(* Logix 5000 Rung export; software revision 33.00 *)

TYPE Banner_IOL_Device_Index_v6 :
STRUCT
   Index : Banner_IOL_Device_SubIndex_v6[41];
END_STRUCT
END_TYPE

TYPE Banner_IOL_Device_SubIndex_v6 :
STRUCT
   Sub : DINT[34];
END_STRUCT
END_TYPE

TYPE Banner_IOL_Device_v6 :
STRUCT
   Initial_Global_Read : BOOL;
   Command : SINT;
   Data : Banner_IOL_Device_Index_v6;
   Reset : BOOL;
END_STRUCT
END_TYPE

TYPE Banner_IOL_Rules_Array_v6 :
STRUCT
   Length : DINT;
   Settings : Banner_IOL_Rules_SettingsArray_v6[41];
END_STRUCT
END_TYPE

TYPE Banner_IOL_Rules_SettingsArray_v6 :
STRUCT
   Index : DINT;
   Sub_Index : DINT;
   Num_Op : INT;   // Number of Operations to read/write Index.
   Total_Bytes : INT;
   RW : SINT;   // 0 = Read Only, 1 = Write Only, 2 = Read or Write
   Rules : Banner_IOL_Rules_v6[34];   // Sub Index Position in IODD.
END_STRUCT
END_TYPE

TYPE Banner_IOL_Rules_v6 :
STRUCT
   Byte_Pos : SINT;   // Byte Position to read from or write data to.
   Multi : SINT;   // Determines if a multiple byte length index is being accessed. Use 2 for 2 bytes length, 3 for 3 byte length, etc..
   BitControl : BOOL;   // 0=Standard byte control, 1=Bitwise packaging
   BitPos : SINT;   // Bit start position for operation
   BitValue : SINT;
   Sub_Index : SINT;
   Signed : SINT;   // 0=Unsigned, 1=Signed
END_STRUCT
END_TYPE

VAR_GLOBAL   (* controller tags *)
   TL70PS_IOLM1_01 : Banner_IOL_Device_v6;
        .DATA.INDEX[2]   // Direct Parameters 1
        .DATA.INDEX[2].SUB[1]   // Reserved
        .DATA.INDEX[2].SUB[2]   // Master Cycle Time
        .DATA.INDEX[2].SUB[3]   // Min Cycle Time
        .DATA.INDEX[2].SUB[4]   // M Sequence Capability
        .DATA.INDEX[2].SUB[5]   // IO-Link Verson ID
        .DATA.INDEX[2].SUB[6]   // Process Data Input Length
        .DATA.INDEX[2].SUB[7]   // Process Data Output Length
        .DATA.INDEX[2].SUB[8]   // Vendor ID
        .DATA.INDEX[2].SUB[9]   // Device ID
        .DATA.INDEX[3]   // Standard Command (wo)
        .DATA.INDEX[3].SUB[1]   // Standard Command: 130=Restore Factory Settings
        .DATA.INDEX[4]   // Device Locks
        .DATA.INDEX[4].SUB[1]   // Parameter Access Lock: 0 to 1
        .DATA.INDEX[4].SUB[2]   // Data Storage Lock: 0 to 1
        .DATA.INDEX[4].SUB[3]   // Local Parameterization Lock: 0 to 1
        .DATA.INDEX[4].SUB[4]   // Local User Interface Lock: 0 to 1
        .DATA.INDEX[5]   // Serial Number (ro)
        .DATA.INDEX[5].SUB[1]   // SN1
        .DATA.INDEX[5].SUB[2]   // SN2
        .DATA.INDEX[5].SUB[3]   // SN3
        .DATA.INDEX[5].SUB[4]   // SN4
        .DATA.INDEX[5].SUB[5]   // SN5
        .DATA.INDEX[5].SUB[6]   // SN6
        .DATA.INDEX[5].SUB[7]   // SN7
        .DATA.INDEX[5].SUB[8]   // SN8
        .DATA.INDEX[5].SUB[9]   // SN9
        .DATA.INDEX[5].SUB[10]   // SN10
        .DATA.INDEX[5].SUB[11]   // SN11
        .DATA.INDEX[5].SUB[12]   // SN12
        .DATA.INDEX[5].SUB[13]   // SN13
        .DATA.INDEX[5].SUB[14]   // SN14
        .DATA.INDEX[5].SUB[15]   // SN15
        .DATA.INDEX[5].SUB[16]   // SN16
        .DATA.INDEX[6]   // Operating Mode Selection
        .DATA.INDEX[6].SUB[1]   // Operating Mode Selection: 0=Basic Segment Mode, 1=Run Mode, 2=Advanced Segment Mode, 3=Level Mode
        .DATA.INDEX[7]   // Segment 1 Configuration
        .DATA.INDEX[7].SUB[1]   // Animation: 0=Off, 1=Steady, 2=Flash, 3=Two Color Flash, 4=Half/Half, 5=Half/Half Rotate, 6=Chase, 7=Intensity Sweep, 8=Demo
        .DATA.INDEX[7].SUB[2]   // Color 1: 0=Green, 1=Red, 2=Orange, 3=Amber, 4=Yellow, 5=Lime Green, 6=Spring Green, 7=Cyan, 8=Sky Blue, 9=Blue, 10=Violet, 11=Magenta, 12=Rose, 13=White
        .DATA.INDEX[7].SUB[3]   // Color 2: 0=Green, 1=Red, 2=Orange, 3=Amber, 4=Yellow, 5=Lime Green, 6=Spring Green, 7=Cyan, 8=Sky Blue, 9=Blue, 10=Violet, 11=Magenta, 12=Rose, 13=White
        .DATA.INDEX[7].SUB[4]   // Color 1 Intensity: 0=High, 1=Medium, 2=Low, 3=Off, 4=Custom
        .DATA.INDEX[7].SUB[5]   // Color 2 Intensity: 0=High, 1=Medium, 2=Low, 3=Off, 4=Custom
        .DATA.INDEX[7].SUB[6]   // Speed: 0=Medium, 1=Slow, 2=Fast, 3=Custom
        .DATA.INDEX[7].SUB[7]   // Pattern: 0=Flash, 1=Strobe, 2=3 Pulse, 3=SOS, 4=Random
        .DATA.INDEX[8]   // Segment 2 Configuration
        .DATA.INDEX[8].SUB[1]   // Animation: 0=Off, 1=Steady, 2=Flash, 3=Two Color Flash, 4=Half/Half, 5=Half/Half Rotate, 6=Chase, 7=Intensity Sweep, 8=Demo
        .DATA.INDEX[8].SUB[2]   // Color 1: 0=Green, 1=Red, 2=Orange, 3=Amber, 4=Yellow, 5=Lime Green, 6=Spring Green, 7=Cyan, 8=Sky Blue, 9=Blue, 10=Violet, 11=Magenta, 12=Rose, 13=White
        .DATA.INDEX[8].SUB[3]   // Color 2: 0=Green, 1=Red, 2=Orange, 3=Amber, 4=Yellow, 5=Lime Green, 6=Spring Green, 7=Cyan, 8=Sky Blue, 9=Blue, 10=Violet, 11=Magenta, 12=Rose, 13=White
        .DATA.INDEX[8].SUB[4]   // Color 1 Intensity: 0=High, 1=Medium, 2=Low, 3=Off, 4=Custom
        .DATA.INDEX[8].SUB[5]   // Color 2 Intensity: 0=High, 1=Medium, 2=Low, 3=Off, 4=Custom
        .DATA.INDEX[8].SUB[6]   // Speed: 0=Medium, 1=Slow, 2=Fast, 3=Custom
        .DATA.INDEX[8].SUB[7]   // Pattern: 0=Flash, 1=Strobe, 2=3 Pulse, 3=SOS, 4=Random
        .DATA.INDEX[9]   // Segment 3 Configuration
        .DATA.INDEX[9].SUB[1]   // Animation: 0=Off, 1=Steady, 2=Flash, 3=Two Color Flash, 4=Half/Half, 5=Half/Half Rotate, 6=Chase, 7=Intensity Sweep, 8=Demo
        .DATA.INDEX[9].SUB[2]   // Color 1: 0=Green, 1=Red, 2=Orange, 3=Amber, 4=Yellow, 5=Lime Green, 6=Spring Green, 7=Cyan, 8=Sky Blue, 9=Blue, 10=Violet, 11=Magenta, 12=Rose, 13=White
        .DATA.INDEX[9].SUB[3]   // Color 2: 0=Green, 1=Red, 2=Orange, 3=Amber, 4=Yellow, 5=Lime Green, 6=Spring Green, 7=Cyan, 8=Sky Blue, 9=Blue, 10=Violet, 11=Magenta, 12=Rose, 13=White
        .DATA.INDEX[9].SUB[4]   // Color 1 Intensity: 0=High, 1=Medium, 2=Low, 3=Off, 4=Custom
        .DATA.INDEX[9].SUB[5]   // Color 2 Intensity: 0=High, 1=Medium, 2=Low, 3=Off, 4=Custom
        .DATA.INDEX[9].SUB[6]   // Speed: 0=Medium, 1=Slow, 2=Fast, 3=Custom
        .DATA.INDEX[9].SUB[7]   // Pattern: 0=Flash, 1=Strobe, 2=3 Pulse, 3=SOS, 4=Random
        .DATA.INDEX[10]   // Segment 4 Configuration
        .DATA.INDEX[10].SUB[1]   // Animation: 0=Off, 1=Steady, 2=Flash, 3=Two Color Flash, 4=Half/Half, 5=Half/Half Rotate, 6=Chase, 7=Intensity Sweep, 8=Demo
        .DATA.INDEX[10].SUB[2]   // Color 1: 0=Green, 1=Red, 2=Orange, 3=Amber, 4=Yellow, 5=Lime Green, 6=Spring Green, 7=Cyan, 8=Sky Blue, 9=Blue, 10=Violet, 11=Magenta, 12=Rose, 13=White
        .DATA.INDEX[10].SUB[3]   // Color 2: 0=Green, 1=Red, 2=Orange, 3=Amber, 4=Yellow, 5=Lime Green, 6=Spring Green, 7=Cyan, 8=Sky Blue, 9=Blue, 10=Violet, 11=Magenta, 12=Rose, 13=White
        .DATA.INDEX[10].SUB[4]   // Color 1 Intensity: 0=High, 1=Medium, 2=Low, 3=Off, 4=Custom
        .DATA.INDEX[10].SUB[5]   // Color 2 Intensity: 0=High, 1=Medium, 2=Low, 3=Off, 4=Custom
        .DATA.INDEX[10].SUB[6]   // Speed: 0=Medium, 1=Slow, 2=Fast, 3=Custom
        .DATA.INDEX[10].SUB[7]   // Pattern: 0=Flash, 1=Strobe, 2=3 Pulse, 3=SOS, 4=Random
        .DATA.INDEX[11]   // Segment 5 Configuration
        .DATA.INDEX[11].SUB[1]   // Animation: 0=Off, 1=Steady, 2=Flash, 3=Two Color Flash, 4=Half/Half, 5=Half/Half Rotate, 6=Chase, 7=Intensity Sweep, 8=Demo
        .DATA.INDEX[11].SUB[2]   // Color 1: 0=Green, 1=Red, 2=Orange, 3=Amber, 4=Yellow, 5=Lime Green, 6=Spring Green, 7=Cyan, 8=Sky Blue, 9=Blue, 10=Violet, 11=Magenta, 12=Rose, 13=White
        .DATA.INDEX[11].SUB[3]   // Color 2: 0=Green, 1=Red, 2=Orange, 3=Amber, 4=Yellow, 5=Lime Green, 6=Spring Green, 7=Cyan, 8=Sky Blue, 9=Blue, 10=Violet, 11=Magenta, 12=Rose, 13=White
        .DATA.INDEX[11].SUB[4]   // Color 1 Intensity: 0=High, 1=Medium, 2=Low, 3=Off, 4=Custom
        .DATA.INDEX[11].SUB[5]   // Color 2 Intensity: 0=High, 1=Medium, 2=Low, 3=Off, 4=Custom
        .DATA.INDEX[11].SUB[6]   // Speed: 0=Medium, 1=Slow, 2=Fast, 3=Custom
        .DATA.INDEX[11].SUB[7]   // Pattern: 0=Flash, 1=Strobe, 2=3 Pulse, 3=SOS, 4=Random
        .DATA.INDEX[12]   // General Config for Level Mode
        .DATA.INDEX[12].SUB[1]   // Full Scale: Number representing Full Scale
        .DATA.INDEX[12].SUB[2]   // Base Color: 0=Green, 1=Red, 2=Orange, 3=Amber, 4=Yellow, 5=Lime Green, 6=Spring Green, 7=Cyan, 8=Sky Blue, 9=Blue, 10=Violet, 11=Magenta, 12=Rose, 13=White
        .DATA.INDEX[12].SUB[3]   // Base Color Intensity: 0=High, 1=Medium, 2=Low, 3=Off, 4=Custom
        .DATA.INDEX[12].SUB[4]   // Base State: 0=Steady, 1=Flashing
        .DATA.INDEX[12].SUB[5]   // Low Threshold: Low Threshold
        .DATA.INDEX[12].SUB[6]   // Low Threshold Color: 0=Green, 1=Red, 2=Orange, 3=Amber, 4=Yellow, 5=Lime Green, 6=Spring Green, 7=Cyan, 8=Sky Blue, 9=Blue, 10=Violet, 11=Magenta, 12=Rose, 13=White
        .DATA.INDEX[12].SUB[7]   // Low Threshold Intensity: 0=High, 1=Medium, 2=Low, 3=Off, 4=Custom
        .DATA.INDEX[12].SUB[8]   // Low Threshold State: 0=Steady, 1=Flashing
        .DATA.INDEX[12].SUB[9]   // High Threshold: High Threshold
        .DATA.INDEX[12].SUB[10]   // High Threshold Color: 0=Green, 1=Red, 2=Orange, 3=Amber, 4=Yellow, 5=Lime Green, 6=Spring Green, 7=Cyan, 8=Sky Blue, 9=Blue, 10=Violet, 11=Magenta, 12=Rose, 13=White
        .DATA.INDEX[12].SUB[11]   // High Threshold Intensity: 0=High, 1=Medium, 2=Low, 3=Off, 4=Custom
        .DATA.INDEX[12].SUB[12]   // High Threshold State: 0=Steady, 1=Flashing
        .DATA.INDEX[12].SUB[13]   // Threshold Type: 0=None, 1=Low, 2=High, 3=Low and High
        .DATA.INDEX[12].SUB[14]   // Flash Rate: 0=Medium, 1=Slow, 2=Fast, 3=Custom
        .DATA.INDEX[12].SUB[15]   // Dominance: 0=NonDominant, 1=Dominant
        .DATA.INDEX[12].SUB[16]   // SubSegment Style: 0=Steady, 1=Flashing, 2=Analog
        .DATA.INDEX[12].SUB[17]   // Background Color: 0=Green, 1=Red, 2=Orange, 3=Amber, 4=Yellow, 5=Lime Green, 6=Spring Green, 7=Cyan, 8=Sky Blue, 9=Blue, 10=Violet, 11=Magenta, 12=Rose, 13=White
        .DATA.INDEX[12].SUB[18]   // Background Color Intensity: 0=High, 1=Medium, 2=Low, 3=Off, 4=Custom
        .DATA.INDEX[12].SUB[19]   // Orientation: 0=Standard, 1=Upside Down
        .DATA.INDEX[13]   // Audible Configuration
        .DATA.INDEX[13].SUB[1]   // Audible Type: 0=Freq, 1=Sync, 2=Off
        .DATA.INDEX[13].SUB[2]   // Volume: 0=High, 1=Medium, 2=Low, 3=Off
        .DATA.INDEX[13].SUB[3]   // Tone 1: 0=Freq 3, 1=Freq 2, 2=Freq 1, 3=Off
        .DATA.INDEX[13].SUB[4]   // Tone 2: 0=Freq 3, 1=Freq 2, 2=Freq 1, 3=Off
        .DATA.INDEX[14]   // Custom Config
        .DATA.INDEX[14].SUB[1]   // Custom Color Intensity (%): 1-255
        .DATA.INDEX[14].SUB[2]   // Custom Animation Speed (dHz): 1-255
   TL70PS_Rules : Banner_IOL_Rules_Array_v6;
        .SETTINGS[2]   // Direct Parameters 1
        .SETTINGS[2].RULES[0]   // Reserved
        .SETTINGS[2].RULES[1]   // Master Cycle Time
        .SETTINGS[2].RULES[2]   // Min Cycle Time
        .SETTINGS[2].RULES[3]   // M-Sequence Capability
        .SETTINGS[2].RULES[4]   // IO-Link ID
        .SETTINGS[2].RULES[5]   // Process Data Input Length
        .SETTINGS[2].RULES[6]   // Process Data Output Length
        .SETTINGS[2].RULES[7]   // Vendor ID
        .SETTINGS[2].RULES[8]   // Device ID
        .SETTINGS[3]   // Standard Command
        .SETTINGS[3].RULES[0]   // Standard Command: 130=Restore Factory Settings
        .SETTINGS[4]   // Device Access Locks
        .SETTINGS[4].RULES[0]   // Parameter Access Lock
        .SETTINGS[4].RULES[1]   // Data Storage Lock
        .SETTINGS[4].RULES[2]   // Local Parameterization Lock
        .SETTINGS[4].RULES[3]   // Local User Interface Lock
        .SETTINGS[5]   // Serial Number
        .SETTINGS[5].RULES[0]   // SN1
        .SETTINGS[5].RULES[1]   // SN2
        .SETTINGS[5].RULES[2]   // SN3
        .SETTINGS[5].RULES[3]   // SN4
        .SETTINGS[5].RULES[4]   // SN5
        .SETTINGS[5].RULES[5]   // SN6
        .SETTINGS[5].RULES[6]   // SN7
        .SETTINGS[5].RULES[7]   // SN8
        .SETTINGS[5].RULES[8]   // SN9
        .SETTINGS[5].RULES[9]   // SN10
        .SETTINGS[5].RULES[10]   // SN11
        .SETTINGS[5].RULES[11]   // SN12
        .SETTINGS[5].RULES[12]   // SN13
        .SETTINGS[5].RULES[13]   // SN14
        .SETTINGS[5].RULES[14]   // SN15
        .SETTINGS[5].RULES[15]   // SN16
        .SETTINGS[6]   // Operating Mode Selection
        .SETTINGS[6].RULES[0]   // Operating Mode Selection: 0=Basic Segment Mode, 1=Run Mode, 2=Advanced Segment Mode, 3=Level Mode
        .SETTINGS[7]   // Segment 1 Configuration
        .SETTINGS[7].RULES[0]   // Animation: 0=Off, 1=Steady, 2=Flash, 3=Two Color Flash, 4=Half/Half, 5=Half/Half Rotate, 6=Chase, 7=Intensity Sweep, 8=Demo
        .SETTINGS[7].RULES[1]   // Color 1: 0=Green, 1=Red, 2=Orange, 3=Amber, 4=Yellow, 5=Lime Green, 6=Spring Green, 7=Cyan, 8=Sky Blue, 9=Blue, 10=Violet, 11=Magenta, 12=Rose, 13=White
        .SETTINGS[7].RULES[2]   // Color 2: 0=Green, 1=Red, 2=Orange, 3=Amber, 4=Yellow, 5=Lime Green, 6=Spring Green, 7=Cyan, 8=Sky Blue, 9=Blue, 10=Violet, 11=Magenta, 12=Rose, 13=White
        .SETTINGS[7].RULES[3]   // Color 1 Intensity: 0=High, 1=Medium, 2=Low, 3=Off, 4=Custom
        .SETTINGS[7].RULES[4]   // Color 2 Intensity: 0=High, 1=Medium, 2=Low, 3=Off, 4=Custom
        .SETTINGS[7].RULES[5]   // Speed: 0=Medium, 1=Slow, 2=Fast, 3=Custom
        .SETTINGS[7].RULES[6]   // Pattern: 0=Flash, 1=Strobe, 2=3 Pulse, 3=SOS, 4=Random
        .SETTINGS[8]   // Segment 2 Configuration
        .SETTINGS[8].RULES[0]   // Animation: 0=Off, 1=Steady, 2=Flash, 3=Two Color Flash, 4=Half/Half, 5=Half/Half Rotate, 6=Chase, 7=Intensity Sweep, 8=Demo
        .SETTINGS[8].RULES[1]   // Color 1: 0=Green, 1=Red, 2=Orange, 3=Amber, 4=Yellow, 5=Lime Green, 6=Spring Green, 7=Cyan, 8=Sky Blue, 9=Blue, 10=Violet, 11=Magenta, 12=Rose, 13=White
        .SETTINGS[8].RULES[2]   // Color 2: 0=Green, 1=Red, 2=Orange, 3=Amber, 4=Yellow, 5=Lime Green, 6=Spring Green, 7=Cyan, 8=Sky Blue, 9=Blue, 10=Violet, 11=Magenta, 12=Rose, 13=White
        .SETTINGS[8].RULES[3]   // Color 1 Intensity: 0=High, 1=Medium, 2=Low, 3=Off, 4=Custom
        .SETTINGS[8].RULES[4]   // Color 2 Intensity: 0=High, 1=Medium, 2=Low, 3=Off, 4=Custom
        .SETTINGS[8].RULES[5]   // Speed: 0=Medium, 1=Slow, 2=Fast, 3=Custom
        .SETTINGS[8].RULES[6]   // Pattern: 0=Flash, 1=Strobe, 2=3 Pulse, 3=SOS, 4=Random
        .SETTINGS[9]   // Segment 3 Configuration
        .SETTINGS[9].RULES[0]   // Animation: 0=Off, 1=Steady, 2=Flash, 3=Two Color Flash, 4=Half/Half, 5=Half/Half Rotate, 6=Chase, 7=Intensity Sweep, 8=Demo
        .SETTINGS[9].RULES[1]   // Color 1: 0=Green, 1=Red, 2=Orange, 3=Amber, 4=Yellow, 5=Lime Green, 6=Spring Green, 7=Cyan, 8=Sky Blue, 9=Blue, 10=Violet, 11=Magenta, 12=Rose, 13=White
        .SETTINGS[9].RULES[2]   // Color 2: 0=Green, 1=Red, 2=Orange, 3=Amber, 4=Yellow, 5=Lime Green, 6=Spring Green, 7=Cyan, 8=Sky Blue, 9=Blue, 10=Violet, 11=Magenta, 12=Rose, 13=White
        .SETTINGS[9].RULES[3]   // Color 1 Intensity: 0=High, 1=Medium, 2=Low, 3=Off, 4=Custom
        .SETTINGS[9].RULES[4]   // Color 2 Intensity: 0=High, 1=Medium, 2=Low, 3=Off, 4=Custom
        .SETTINGS[9].RULES[5]   // Speed: 0=Medium, 1=Slow, 2=Fast, 3=Custom
        .SETTINGS[9].RULES[6]   // Pattern: 0=Flash, 1=Strobe, 2=3 Pulse, 3=SOS, 4=Random
        .SETTINGS[10]   // Segment 4 Configuration
        .SETTINGS[10].RULES[0]   // Animation: 0=Off, 1=Steady, 2=Flash, 3=Two Color Flash, 4=Half/Half, 5=Half/Half Rotate, 6=Chase, 7=Intensity Sweep, 8=Demo
        .SETTINGS[10].RULES[1]   // Color 1: 0=Green, 1=Red, 2=Orange, 3=Amber, 4=Yellow, 5=Lime Green, 6=Spring Green, 7=Cyan, 8=Sky Blue, 9=Blue, 10=Violet, 11=Magenta, 12=Rose, 13=White
        .SETTINGS[10].RULES[2]   // Color 2: 0=Green, 1=Red, 2=Orange, 3=Amber, 4=Yellow, 5=Lime Green, 6=Spring Green, 7=Cyan, 8=Sky Blue, 9=Blue, 10=Violet, 11=Magenta, 12=Rose, 13=White
        .SETTINGS[10].RULES[3]   // Color 1 Intensity: 0=High, 1=Medium, 2=Low, 3=Off, 4=Custom
        .SETTINGS[10].RULES[4]   // Color 2 Intensity: 0=High, 1=Medium, 2=Low, 3=Off, 4=Custom
        .SETTINGS[10].RULES[5]   // Speed: 0=Medium, 1=Slow, 2=Fast, 3=Custom
        .SETTINGS[10].RULES[6]   // Pattern: 0=Flash, 1=Strobe, 2=3 Pulse, 3=SOS, 4=Random
        .SETTINGS[11]   // Segment 5 Configuration
        .SETTINGS[11].RULES[0]   // Animation: 0=Off, 1=Steady, 2=Flash, 3=Two Color Flash, 4=Half/Half, 5=Half/Half Rotate, 6=Chase, 7=Intensity Sweep, 8=Demo
        .SETTINGS[11].RULES[1]   // Color 1: 0=Green, 1=Red, 2=Orange, 3=Amber, 4=Yellow, 5=Lime Green, 6=Spring Green, 7=Cyan, 8=Sky Blue, 9=Blue, 10=Violet, 11=Magenta, 12=Rose, 13=White
        .SETTINGS[11].RULES[2]   // Color 2: 0=Green, 1=Red, 2=Orange, 3=Amber, 4=Yellow, 5=Lime Green, 6=Spring Green, 7=Cyan, 8=Sky Blue, 9=Blue, 10=Violet, 11=Magenta, 12=Rose, 13=White
        .SETTINGS[11].RULES[3]   // Color 1 Intensity: 0=High, 1=Medium, 2=Low, 3=Off, 4=Custom
        .SETTINGS[11].RULES[4]   // Color 2 Intensity: 0=High, 1=Medium, 2=Low, 3=Off, 4=Custom
        .SETTINGS[11].RULES[5]   // Speed: 0=Medium, 1=Slow, 2=Fast, 3=Custom
        .SETTINGS[11].RULES[6]   // Pattern: 0=Flash, 1=Strobe, 2=3 Pulse, 3=SOS, 4=Random
        .SETTINGS[12]   // General Config for Level Mode
        .SETTINGS[12].RULES[0]   // Full Scale: Number representing Full Scale
        .SETTINGS[12].RULES[1]   // Base Color: 0=Green, 1=Red, 2=Orange, 3=Amber, 4=Yellow, 5=Lime Green, 6=Spring Green, 7=Cyan, 8=Sky Blue, 9=Blue, 10=Violet, 11=Magenta, 12=Rose, 13=White
        .SETTINGS[12].RULES[2]   // Base Color Intensity: 0=High, 1=Medium, 2=Low, 3=Off, 4=Custom
        .SETTINGS[12].RULES[3]   // Base State: 0=Steady, 1=Flashing
        .SETTINGS[12].RULES[4]   // Low Threshold: Low Threshold
        .SETTINGS[12].RULES[5]   // Low Threshold Color: 0=Green, 1=Red, 2=Orange, 3=Amber, 4=Yellow, 5=Lime Green, 6=Spring Green, 7=Cyan, 8=Sky Blue, 9=Blue, 10=Violet, 11=Magenta, 12=Rose, 13=White
        .SETTINGS[12].RULES[6]   // Low Threshold Intensity: 0=High, 1=Medium, 2=Low, 3=Off, 4=Custom
        .SETTINGS[12].RULES[7]   // Low Threshold State: 0=Steady, 1=Flashing
        .SETTINGS[12].RULES[8]   // High Threshold: High Threshold
        .SETTINGS[12].RULES[9]   // High Threshold Color: 0=Green, 1=Red, 2=Orange, 3=Amber, 4=Yellow, 5=Lime Green, 6=Spring Green, 7=Cyan, 8=Sky Blue, 9=Blue, 10=Violet, 11=Magenta, 12=Rose, 13=White
        .SETTINGS[12].RULES[10]   // High Threshold Intensity: 0=High, 1=Medium, 2=Low, 3=Off, 4=Custom
        .SETTINGS[12].RULES[11]   // High Threshold State: 0=Steady, 1=Flashing
        .SETTINGS[12].RULES[12]   // Threshold Type: 0=None, 1=Low, 2=High, 3=Low and High
        .SETTINGS[12].RULES[13]   // Flash Rate: 0=Medium, 1=Slow, 2=Fast, 3=Custom
        .SETTINGS[12].RULES[14]   // Dominance: 0=NonDominant, 1=Dominant
        .SETTINGS[12].RULES[15]   // SubSegment Style: 0=Steady, 1=Flashing, 2=Analog
        .SETTINGS[12].RULES[16]   // Background Color: 0=Green, 1=Red, 2=Orange, 3=Amber, 4=Yellow, 5=Lime Green, 6=Spring Green, 7=Cyan, 8=Sky Blue, 9=Blue, 10=Violet, 11=Magenta, 12=Rose, 13=White
        .SETTINGS[12].RULES[17]   // Background Color Intensity: 0=High, 1=Medium, 2=Low, 3=Off, 4=Custom
        .SETTINGS[12].RULES[18]   // Orientation: 0=Standard, 1=Upside Down
        .SETTINGS[13]   // Audible Configuration
        .SETTINGS[13].RULES[0]   // Audible Type: 0=Freq, 1=Sync, 2=Off
        .SETTINGS[13].RULES[1]   // Volume: 0=High, 1=Medium, 2=Low, 3=Off
        .SETTINGS[13].RULES[2]   // Tone 1: 0=Freq 3, 1=Freq 2, 2=Freq 1, 3=Off
        .SETTINGS[13].RULES[3]   // Tone 2: 0=Freq 3, 1=Freq 2, 2=Freq 1, 3=Off
        .SETTINGS[14]   // Custom Config
        .SETTINGS[14].RULES[0]   // Custom Color Intensity (%): 1-255
        .SETTINGS[14].RULES[1]   // Custom Animation Speed (dHz): 1-255
END_VAR

PROGRAM MainProgram

ROUTINE MainRoutine   (* ladder *)
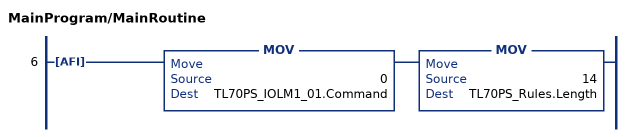
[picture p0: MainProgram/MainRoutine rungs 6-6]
   6: AFI()MOV(0,TL70PS_IOLM1_01.Command)MOV(14,TL70PS_Rules.Length);
END_ROUTINE
END_PROGRAM
